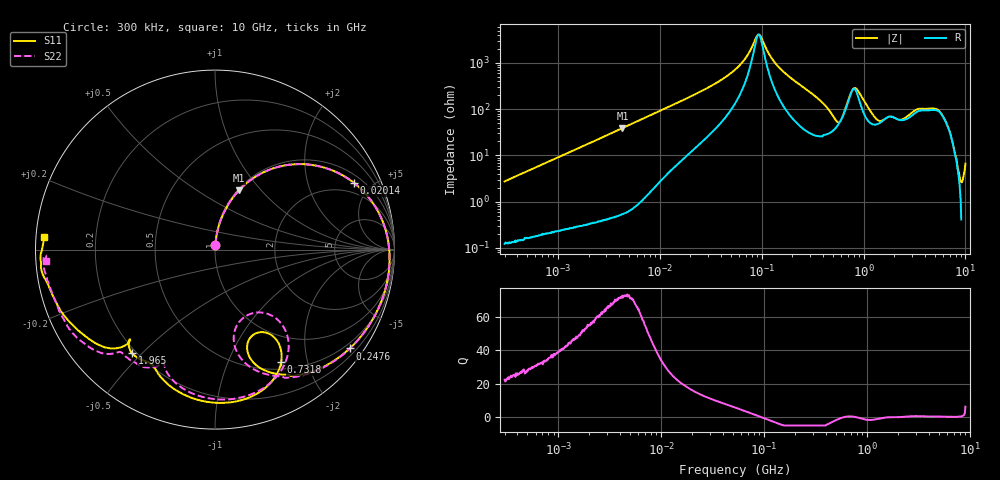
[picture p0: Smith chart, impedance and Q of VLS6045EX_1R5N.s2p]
! S-Parameter Data Generated by TDK Corporation
! Copyright(C) 2019 TDK Corporation.
! All Rights Reserved.
! TDK P/N: VLS6045EX-1R5N (Inductor)
! Property: L=1.5uH at 100kHz
! Size(LxWxT): 6x6x4.5mm
! Model Type: s2p (Touchstone File Format Version 1.0)
! Frequency: DC=Yes Start=0.3MHz Stop=10000MHz 802points Log-sweep
! Model Generated on May 10, 2019
! Port Assignments:
!  1 ---@@@--- 2
! Applicable Conditions:
!  Temperature = 25 degC
!  DC Bias Current = 0 A
!  Small Signal Operation
! Terms and conditions regarding TDK Simulation Models
! (1)This simulation model is being provided solely for informational purposes. Please refer to the specifications of the products in terms of detailed characteristics of such products.
! (2)In no event shall TDK Corporation of any of its subsidiaries be liable for any loss or damage arising, directly or indirectly,
!  From any information contained in this simulation model, including, but not limited to loss or damages arising from any inaccuracies, omissions or errors in connection with such information.
! (3)Any and all copyrights on this simulation model are owned by TDK Corporation.
!  Duplication or redistribution of this simulation model without prior written permission from TDK Corporation is prohibited.
! (4)This simulation model is subject to any modification or change without any prior notice.
! (5)Neither TDK Corporation nor any of its subsidiaries shall make any warranty, express or implied,
!  Including but not limited to the correctness, implied warranties of merchantability and fitness for a particular purpose with respect to this simulation models.
! (6)The use of this simulation model shall be deemed to have consented to the terms and conditions hereof.
# Hz S MA R 50
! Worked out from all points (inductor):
!   801 points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, 300 kHz to 10 GHz, reference 50 ohm
!   read as one part in series: L = 1.45 uH near 318.3 kHz
!   highest Q = 72.5 at 4.301 MHz (marker M1), where L = 1.43 uH
!   self-resonance near 93.68 MHz
!   S11 on the Smith chart (normalised r, x): 300 kHz: 1.00, +0.05; 20.14 MHz: 1.38, +3.93; 247.6 MHz: 0.37, -3.02; 731.8 MHz: 0.59, -1.58; 1.965 GHz: 0.18, -0.47; 10 GHz: 0.02, +0.04
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300000  0.02653 86.1  0.9983 -1.6  0.9985 -1.6  0.02632 85.5
1713600  0.1505 80.1  0.9856 -8.8  0.9858 -8.8  0.1505 80.0
4301371  0.3561 68.0  0.9294 -21.2  0.9295 -21.2  0.3562 68.0
9671944  0.6486 47.1  0.743 -41.2  0.743 -41.2  0.6486 47.1
2.013744e7  0.8591 25.6  0.4605 -60.8  0.4605 -60.8  0.8591 25.6
5.477226e7  0.9655 3.1  0.1364 -76.3  0.1365 -76.3  0.9655 2.9
9.444554e7  0.9763 -8.1  0.02367 -3.3  0.02368 -3.3  0.9763 -8.3
1.454054e8  0.969 -18.6  0.1133 58.6  0.1133 58.6  0.9688 -19.0
2.476102e8  0.9308 -36.2  0.2709 46.4  0.2708 46.4  0.9295 -37.1
3.126428e8  0.8935 -46.5  0.3567 36.0  0.3567 36.0  0.8904 -47.9
5.285151e8  0.6197 -72.3  0.5789 -10.2  0.5789 -10.2  0.5701 -78.2
6.325141e8  0.5346 -59.4  0.5177 -43.6  0.5176 -43.6  0.4193 -56.8
7.318083e8  0.7282 -59.6  0.2927 -61.0  0.2926 -60.9  0.6624 -51.8
8.299813e8  0.8316 -72.5  0.1929 -39.4  0.1929 -39.4  0.7983 -66.2
9.789263e8  0.8545 -88.9  0.2578 -22.2  0.2578 -22.2  0.8381 -84.3
1.339606e9  0.7735 -112.8  0.3653 -47.8  0.3656 -47.8  0.7474 -110.0
1.767019e9  0.7367 -123.1  0.2866 -80.6  0.2869 -80.7  0.7249 -116.3
1.964718e9  0.739 -128.6  0.2572 -85.6  0.2574 -85.7  0.7689 -121.8
2.629198e9  0.6932 -133.0  0.2133 -117.3  0.213 -117.5  0.7839 -133.2
5.76861e9  0.9306 -161.1  0.03842 -149.6  0.03832 -149.2  0.9305 -157.6
8.322921e9  0.9733 -176.4  0.02415 -144.4  0.02432 -143.9  0.9575 -175.9
1e10  0.953 175.7  0.02754 -136.6  0.02765 -136.6  0.9439 -176.2
